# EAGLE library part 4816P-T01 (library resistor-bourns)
BOURNS RESISTOR NETWORK
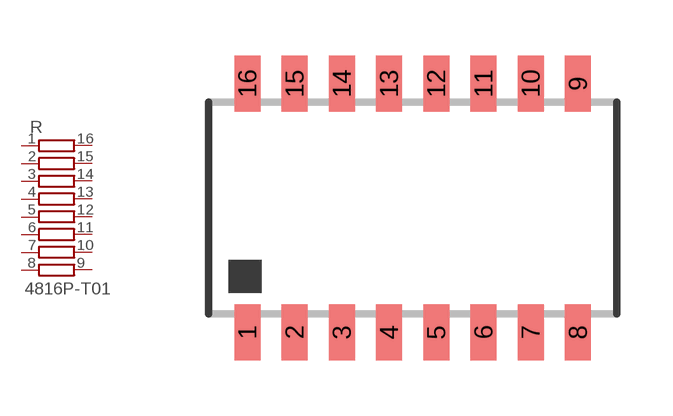
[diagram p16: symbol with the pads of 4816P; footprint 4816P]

Designator prefix R

## 4816P-T01 (MF: BOURNS, INC.; MPN: 4816P-T01-684LF; OC_FARNELL: 9357483; OC_NEWARK: 33K0707)  [4816P]
1  1  pas
2  2  pas
3  3  pas
4  4  pas
5  5  pas
6  6  pas
7  7  pas
8  8  pas
9  9  pas
10  10  pas
11  11  pas
12  12  pas
13  13  pas
14  14  pas
15  15  pas
16  16  pas

## Footprint 4816P (pad centres in mm)
BOURNS RESISTOR NETWORK
smd 0.7 x 1.5: 1 -4.445,-3.346; 2 -3.175,-3.346; 3 -1.905,-3.346; 4 -0.635,-3.346; 5 0.635,-3.346; 6 1.905,-3.346; 7 3.175,-3.346; 8 4.445,-3.346; 9 4.445,3.346; 10 3.175,3.346; 11 1.905,3.346; 12 0.635,3.346; 13 -0.635,3.346; 14 -1.905,3.346; 15 -3.175,3.346; 16 -4.445,3.346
